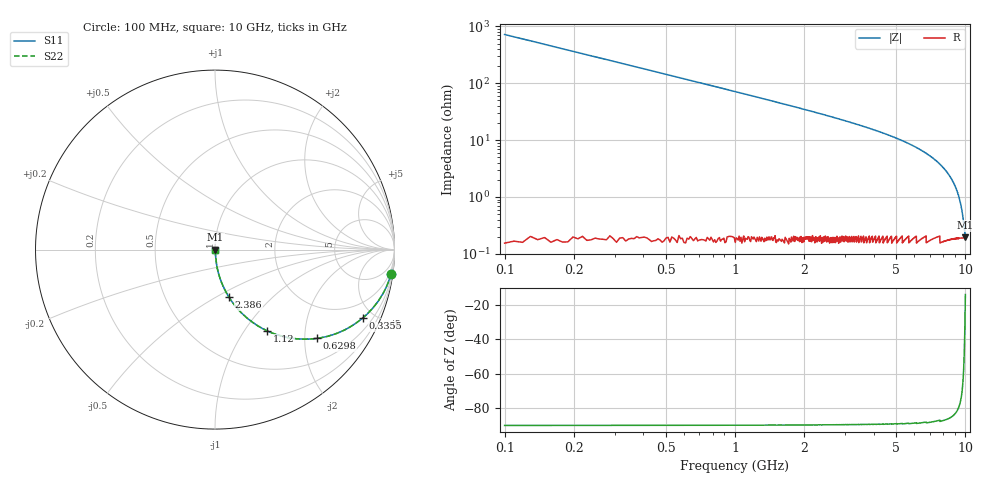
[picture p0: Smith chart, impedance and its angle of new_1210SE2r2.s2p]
!	AVX	Thin	Film	Operation	Date:	April 2007
!	Description:	Accu-P®	"Series,"	Thin	"Film,"	"SMD,"	RF	Capacitor
!	Part	Number:	12101J2R2ABT
!	100	MHz	-	6.05	GHz
!	Serial	Measurements
#	MHZ	S	MA	R	50
!	S11	S21	S12	S22
!	dB	Phase	dB	Phase	dB	Phase	dB	Phase
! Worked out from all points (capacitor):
!   1010 points, 100 MHz to 10 GHz, reference 50 ohm
!   read as one part in series: C = 2.2 pF near 149.1 MHz
!   lowest |Z| = 196 mohm at 10 GHz (marker M1)
!   S11 on the Smith chart (normalised r, x): 100 MHz: 1, -14; 335.5 MHz: 1.00, -4.31; 629.8 MHz: 1.00, -2.29; 1.12 GHz: 1.00, -1.28; 2.386 GHz: 1.00, -0.57; 10 GHz: 1.00, -0.00
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100  0.991 -7.9  0.137 82.1  0.137 82.1  0.991 -7.9
217.74  0.957 -16.8  0.288 73.2  0.288 73.2  0.957 -16.8
335.481  0.907 -24.9  0.421 65.1  0.421 65.1  0.907 -24.9
463.033  0.841 -32.7  0.54 57.3  0.54 57.3  0.841 -32.7
629.832  0.752 -41.1  0.658 48.8  0.658 48.8  0.752 -41.1
865.312  0.638 -50.2  0.769 39.6  0.769 39.6  0.638 -50.2
1120.416  0.537 -57.4  0.842 32.5  0.842 32.5  0.537 -57.4
1404.955  0.45 -63.1  0.891 26.7  0.891 26.7  0.45 -63.1
1758.176  0.37 -68.0  0.927 21.7  0.927 21.7  0.37 -68.0
2386.125  0.275 -73.7  0.96 15.9  0.96 15.9  0.275 -73.7
3406.541  0.184 -78.8  0.981 10.6  0.981 10.6  0.184 -78.8
5054.906  0.106 -83.0  0.993 6.1  0.993 6.1  0.106 -83.0
6703.271  0.06 -84.9  0.996 3.4  0.996 3.4  0.06 -84.9
7547.076  0.042 -85.1  0.997 2.4  0.997 2.4  0.042 -85.1
8351.635  0.027 -84.6  0.998 1.5  0.998 1.5  0.027 -84.6
8901.09  0.017 -83.1  0.998 1.0  0.998 1.0  0.017 -83.1
9215.064  0.012 -81.0  0.998 0.7  0.998 0.7  0.012 -81.0
9421.11  0.00923 -78.3  0.998 0.5  0.998 0.5  0.00923 -78.3
9695.837  0.00523 -69.6  0.998 0.3  0.998 0.3  0.00523 -69.6
9803.766  0.00377 -61.4  0.998 0.2  0.998 0.2  0.00377 -61.4
9950.942  0.00215 -33.1  0.998 0.1  0.998 0.1  0.00215 -33.1
10000  0.00186 -14.5  0.998 0.0  0.998 0.0  0.00186 -14.5
